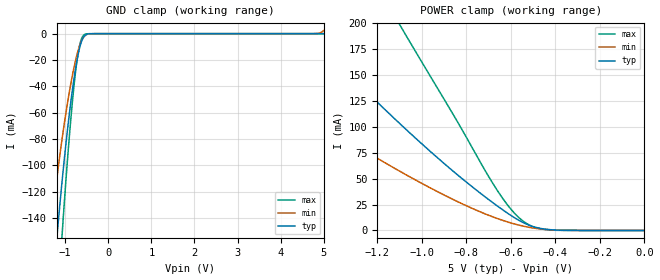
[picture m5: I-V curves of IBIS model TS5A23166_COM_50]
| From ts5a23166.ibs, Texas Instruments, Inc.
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[Model]   TS5A23166_COM_50
Model_type  Terminator
| variable   typ   min   max
C_comp   24.45pF   17.26pF   39.26pF
| C_tri-state   24.45pF   17.26pF   39.26pF
[Temperature Range]   40   100   -40
| Ambient temperature   25   85   -40
[Voltage range]   5   4.5   5.5
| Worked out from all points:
|   GND clamp passes 1 mA (typ) near -0.52 V on its own axis
|   POWER clamp passes 1 mA (typ) near -0.43 V on its own axis
[GND Clamp]
| TS5A23166_COM_50
|   Voltage   I(typ)   I(min)   I(max)
-5V       -2.406A    -1.84A     -3.08A
-1.35V    -217.1mA   -153.4mA   -304mA
-1.31V    -200.7mA   -141.9mA   -280.7mA
-1.185V   -152.3mA   -108mA     -211.2mA
-1.065V   -110.1mA   -78.58mA   -150mA
-900mV    -60.24mA   -43.85mA   -77.18mA
-770mV    -28.93mA   -21.99mA   -32.19mA
-720mV    -19.34mA   -15.24mA   -19.35mA
-655mV    -9.64mA    -8.219mA   -7.662mA
-535mV    -1.224mA   -1.366mA   -440.9uA
4.775V    216.6pA    23.68uA    117.7pA
5V        1.641nA    2.424mA    126.3pA
[POWER Clamp]
| TS5A23166_COM_50
|   Voltage   I(typ)   I(min)   I(max)
-5V       1.304A     844.3mA    2.188A
-2.04V    320.1mA    191.9mA    580.8mA
-1.535V   197.4mA    114.9mA    366.8mA
-1.5V     189.4mA    109.9mA    352.7mA
-1.12V    107.6mA    59.84mA    206.5mA
-1.065V   96.52mA    53.17mA    186.4mA
-680mV    26.77mA    13.08mA    45.27mA
-610mV    16.05mA    7.933mA    23.41mA
-545mV    7.685mA    4.25mA     9.112mA
-495mV    3.446mA    2.259mA    3.203mA
-425mV    793.9uA    694uA      469.8uA
-84.45fV  1.641nA    9.572nA    173.9pA
